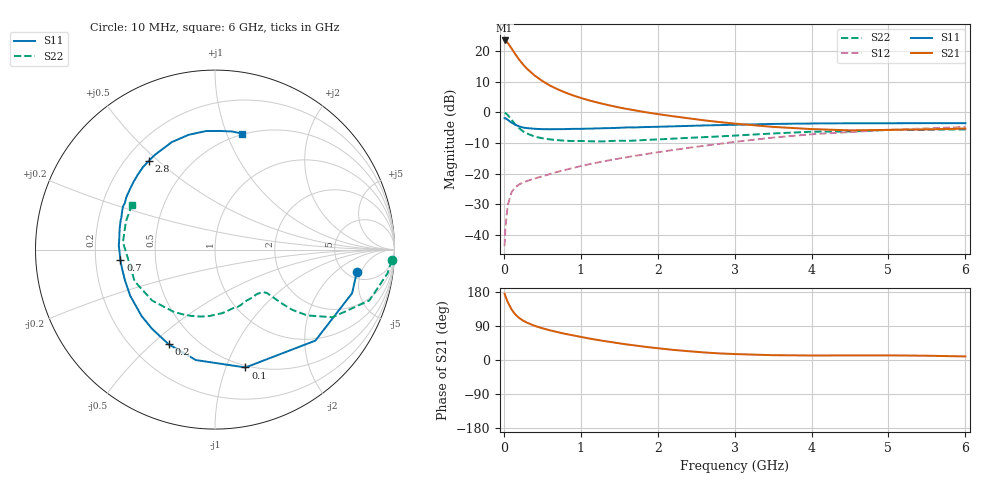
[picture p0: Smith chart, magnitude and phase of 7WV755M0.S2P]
! Infineon Technologies  Discrete & RF Semiconductors
! BFS17W
! Si NPN RF Bipolar Junction Transistor in SOT323
! VCE = 0.75 V  IC = 5 mA
! Common Emitter S-Parameters:  August  1999
# GHz  S  MA  R  50
!  f  S11  S21  S12  S22
! GHz  MAG  ANG  MAG  ANG  MAG  ANG  MAG  ANG
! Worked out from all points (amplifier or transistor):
!   36 points, 10 MHz to 6 GHz, reference 50 ohm
!   highest |S21| = 23.5 dB at 10 MHz (marker M1)
!   |S21| within 3 dB of that: start of sweep to 110.7 MHz
!   unconditionally stable (mu >= 1): 478.2 MHz to end of sweep
!   at 250 MHz: K = 0.63, MSG = 19.3 dB, |S12| = -22.9 dB
!   at 1.4 GHz: K = 1.36, MAG = 5.2 dB, |S12| = -15.6 dB
!   at 6 GHz: K = 1.13, MAG = -2.5 dB, |S12| = -4.8 dB
!   S11 on the Smith chart (normalised r, x): 10 MHz: 6.12, -4.16; 100 MHz: 0.48, -1.17; 200 MHz: 0.35, -0.57; 700 MHz: 0.31, -0.05; 2.8 GHz: 0.29, +0.47; 6 GHz: 0.49, +1.13
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0.01  0.8001 -8.8  14.91 175.0  0.0065 84.1  0.9866 -3.5
0.02  0.8017 -17.6  14.75 168.9  0.0128 80.3  0.9706 -7.8
0.05  0.7549 -42.2  13.65 153.2  0.0301 70.2  0.9057 -18.2
0.1  0.6783 -75.5  11.07 133.6  0.0496 55.4  0.7562 -29.9
0.15  0.6246 -99.8  8.86 119.9  0.0598 47.3  0.6316 -35.5
0.2  0.5872 -116.1  7.226 110.8  0.0663 44.5  0.5477 -37.9
0.25  0.5636 -128.6  6.035 104.0  0.0714 42.1  0.4883 -38.7
0.3  0.5517 -137.8  5.162 98.6  0.0753 42.0  0.4504 -39.1
0.4  0.5379 -151.5  3.991 90.2  0.0827 42.7  0.4011 -39.6
0.5  0.5302 -160.8  3.249 83.8  0.0899 44.4  0.3769 -39.9
0.6  0.5284 -167.7  2.731 78.3  0.0981 46.3  0.3606 -41.2
0.7  0.5304 -173.5  2.376 73.5  0.1069 47.9  0.3506 -43.2
0.9  0.5364 177.6  1.886 65.0  0.1232 50.3  0.3388 -48.2
1.1  0.5406 169.9  1.576 57.1  0.141 51.8  0.3364 -54.4
1.3  0.5496 163.2  1.361 50.2  0.1584 52.8  0.3351 -61.5
1.6  0.566 155.0  1.134 41.1  0.1847 53.4  0.3415 -72.3
2.2  0.5895 140.6  0.862 26.7  0.242 53.8  0.3713 -94.8
2.8  0.6173 126.7  0.693 17.4  0.3048 51.4  0.4035 -116.9
3.5  0.6455 112.0  0.577 12.7  0.3859 46.0  0.4509 -141.0
4.5  0.6624 94.3  0.507 12.1  0.4747 34.6  0.4859 -173.1
5.5  0.6649 81.7  0.525 11.3  0.5464 24.2  0.5205 162.6
6  0.6635 76.9  0.543 9.4  0.5763 19.1  0.5253 152.0
